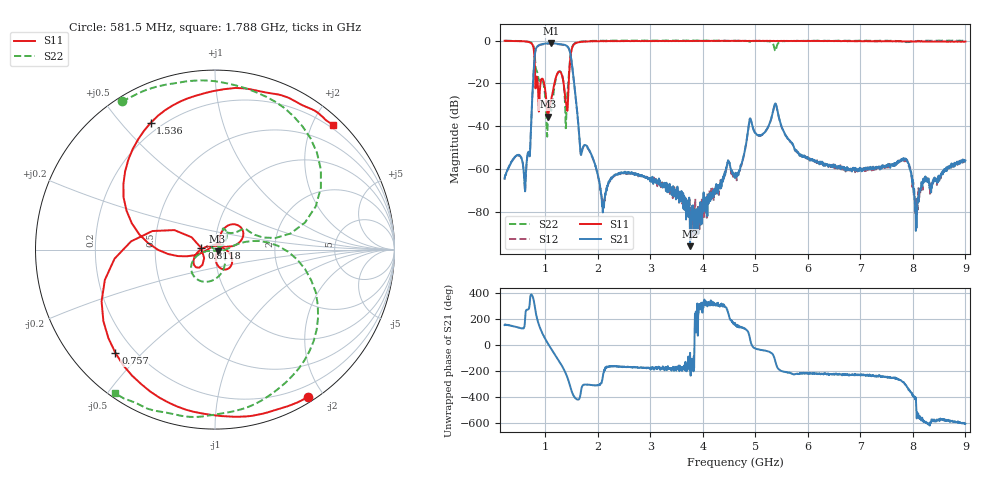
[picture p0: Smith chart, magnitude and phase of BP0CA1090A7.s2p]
!Agilent Technologies,E8358A,US41080443,A.07.50.56
!Agilent E8358A: A.07.50.56
!Date: Thursday, November 09, 2017 08:33:41
!Correction: S11(Full 2 Port(1,2))
!S21(Full 2 Port(1,2))
!S12(Full 2 Port(1,2))
!S22(Full 2 Port(1,2))
!S2P File: Measurements: S11, S21, S12, S22:
# Hz S  dB  R 50
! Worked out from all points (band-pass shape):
!   1601 points, 225 MHz to 9 GHz, reference 50 ohm
!   highest |S21| = -1.23 dB at 1.103 GHz (marker M1); lowest = -96.1 dB at 3.757 GHz (marker M2)
!   |S21| within 3 dB of the highest: 815.8 MHz to 1.458 GHz (642.2 MHz wide, 56.5 % of centre)
!   lowest |S11| = -35.5 dB at 1.048 GHz (marker M3), VSWR 1.03, Z = 51.4 - j0.949 ohm
!   |S11| at or under -10 dB: 797.5 MHz to 1.47 GHz (672.4 MHz wide, 59.3 % of centre)
!   |S22| runs from -44.9 to 0.1 dB; largest |S21 - S12| = 0.016
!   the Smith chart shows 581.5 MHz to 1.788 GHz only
!   S11 on the Smith chart (normalised r, x): 581.5 MHz: 0.07, -1.81; 757 MHz: 0.13, -0.42; 811.8 MHz: 0.86, +0.01; 1.536 GHz: 0.16, +0.60; 1.788 GHz: 0.14, +2.31
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2.25e8  -0.06 -16.2  -64.45 155.0  -65.02 156.6  -0.01 163.1
5.814844e8  -0.27 -57.9  -58.99 128.8  -59.20 127.5  -0.21 122.2
7.569844e8  -1.94 -134.0  -23.86 17.3  -23.98 17.2  -1.29 59.4
8.118281e8  -22.31 173.7  -4.63 -93.5  -4.77 -93.4  -11.17 14.0
9.379688e8  -17.75 -51.6  -1.63 96.0  -1.78 96.2  -18.16 62.4
1.047656e9  -35.49 -33.3  -1.26 12.8  -1.41 13.0  -37.38 146.7
1.1025e9  -28.66 42.9  -1.23 -23.1  -1.38 -23.0  -32.27 92.7
1.327359e9  -17.02 16.2  -1.76 -168.5  -1.91 -168.4  -16.83 -151.3
1.404141e9  -30.14 74.4  -2.37 126.4  -2.50 126.4  -31.14 -16.4
1.535766e9  -2.02 116.9  -16.95 -29.7  -17.11 -30.0  -1.81 -55.1
1.689328e9  -0.54 61.8  -52.67 26.1  -52.88 26.1  -0.42 -108.6
1.788047e9  -0.38 46.7  -49.15 53.1  -49.42 52.6  -0.25 -124.8
2.100656e9  -0.26 20.8  -77.15 123.7  -77.38 138.5  -0.01 -144.0
3.153656e9  -0.17 -18.6  -65.28 -177.6  -67.17 -174.9  0.11 -166.4
3.756938e9  -0.09 -30.7  -96.13 -60.7  -77.72 -177.3  0.05 -174.2
4.6125e9  -0.06 -41.4  -64.24 170.6  -62.47 153.5  -0.02 171.0
5.374828e9  -0.17 -48.5  -29.48 -116.8  -29.54 -116.8  -4.70 148.0
6.076828e9  -0.12 -56.1  -55.36 137.7  -56.42 140.0  -0.09 137.8
7.541156e9  -0.32 -83.5  -58.60 108.1  -58.88 112.0  -0.10 114.1
7.886672e9  -0.32 -92.9  -56.29 34.3  -55.69 41.1  -0.64 112.1
8.073141e9  -0.38 -98.3  -79.81 152.3  -76.91 -164.7  -0.22 113.8
9e9  -0.41 -126.1  -56.04 112.0  -56.37 109.9  -0.02 106.3
